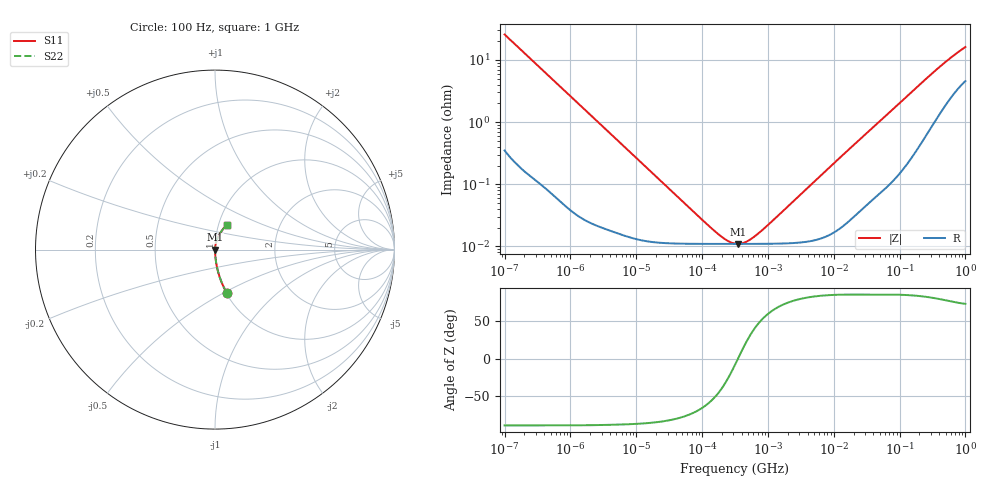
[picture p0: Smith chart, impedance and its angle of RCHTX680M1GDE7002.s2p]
! RCHTX680M1GDE7002  S-PARAMETER MODEL  (AEC-Q200 qualified)
! Model Generated by ELNA Corporation (http://www.ty-top.com)
! Version 1.0
! ELNA Control No.231201
! Copyright (c) 2023 ELNA CO.,LTD. All Rights Reserved.
! Products Name : CONDUCTIVE POLYMER HYBRID ALUMINUM ELECTROLYTIC CAPACITORS
! Characteristics :
!  Capacitance  :  68uF  ,  Rated voltage  :  35V
!  Operating Temp. Range  :  -55 to +135 degC  ,  Endurance  :  2000hr at 135 degC
!  Dimension D  :  6.3mm  ,  Dimension L  :  7.7mm
! Frequency Range : 100Hz - 1GHz
! External Node Assignments :
!  1  o---| |---o  2
# MHz S RI R 50
!Freq[MHz].  S11 Real  S11 Imag  S21 Real  S21 Imag  S12 Real  S12 Imag  S22 Real  S22 Imag
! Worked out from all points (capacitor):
!   401 points, 100 Hz to 1 GHz, reference 50 ohm
!   read as one part in series: C = 61.7 uF near 108 Hz
!   lowest |Z| = 10.9 mohm at 356.9 kHz (marker M1)
!   series resonance near 350.2 kHz, so ESL is about 3.3 nH
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0.0001  0.0651 -0.24  0.9349 0.24  0.9349 0.24  0.0651 -0.24
0.000113  0.0521 -0.2158  0.9479 0.2158  0.9479 0.2158  0.0521 -0.2158
0.000183  0.0211 -0.1378  0.9789 0.1378  0.9789 0.1378  0.0211 -0.1378
0.000309  0.00806 -0.083  0.9919 0.083  0.9919 0.083  0.00806 -0.083
0.000613  0.0024 -0.0423  0.9976 0.0423  0.9976 0.0423  0.0024 -0.0423
0.001488  0.000591 -0.0176  0.9994 0.0176  0.9994 0.0176  0.000591 -0.0176
0.022131  0.000116 -0.0012  0.9999 0.0012  0.9999 0.0012  0.000116 -0.0012
0.094406  0.00011 -0.000262  0.9999 0.000262  0.9999 0.000262  0.00011 -0.000262
0.165959  0.000109 -0.000124  0.9999 0.000124  0.9999 0.000124  0.000109 -0.000124
0.238506  0.000109 -5.99e-05  0.9999 5.99e-05  0.9999 5.99e-05  0.000109 -5.99e-05
0.316228  0.000109 -1.55e-05  0.9999 1.55e-05  0.9999 1.55e-05  0.000109 -1.55e-05
0.356862  0.000109 2.91e-06  0.9999 -2.91e-06  0.9999 -2.91e-06  0.000109 2.91e-06
0.419276  0.000109 2.76e-05  0.9999 -2.76e-05  0.9999 -2.76e-05  0.000109 2.76e-05
0.492606  0.000109 5.3e-05  0.9999 -5.3e-05  0.9999 -5.3e-05  0.000109 5.3e-05
0.707946  0.000109 0.000116  0.9999 -0.000116  0.9999 -0.000116  0.000109 0.000116
1.195364  0.00011 0.000237  0.9999 -0.000237  0.9999 -0.000237  0.00011 0.000237
4.704354  0.000124 0.00102  0.9999 -0.00102  0.9999 -0.00102  0.000124 0.00102
69.9842  0.00118 0.0142  0.9988 -0.0142  0.9988 -0.0142  0.00118 0.0142
176.8072  0.00457 0.0348  0.9954 -0.0348  0.9954 -0.0348  0.00457 0.0348
380.1894  0.0169 0.07  0.9831 -0.07  0.9831 -0.07  0.0169 0.07
668.3439  0.0399 0.1078  0.9601 -0.1078  0.9601 -0.1078  0.0399 0.1078
1000  0.0645 0.1392  0.9355 -0.1392  0.9355 -0.1392  0.0645 0.1392
